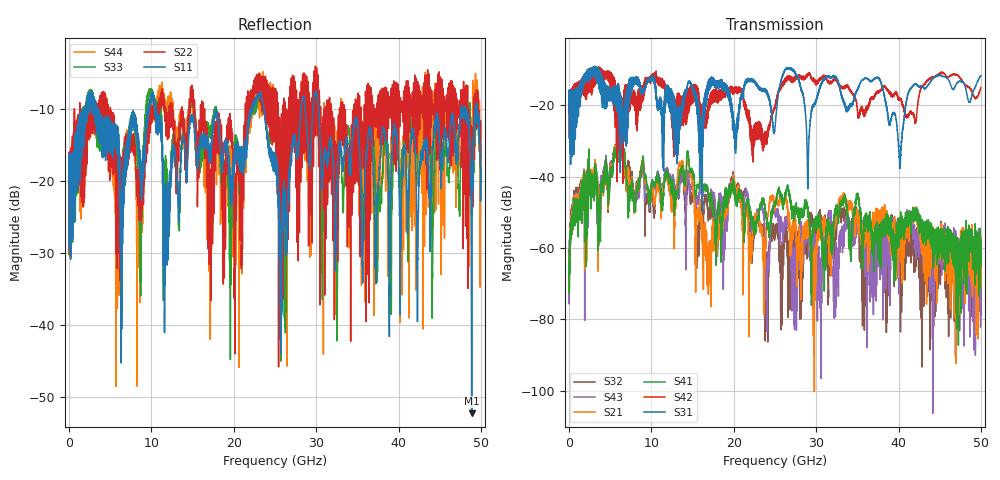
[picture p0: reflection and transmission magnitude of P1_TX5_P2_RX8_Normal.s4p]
!Keysight Technologies,N5225B,MY57041031,A.13.20.10
!Date: Friday, May 31, 2019 11:40:32
!Correction: S11(Full 4 Port(1,2,3,4))
!S12(Full 4 Port(1,2,3,4))
!S13(Full 4 Port(1,2,3,4))
!S14(Full 4 Port(1,2,3,4))
!S21(Full 4 Port(1,2,3,4))
!S22(Full 4 Port(1,2,3,4))
!S23(Full 4 Port(1,2,3,4))
!S24(Full 4 Port(1,2,3,4))
!S31(Full 4 Port(1,2,3,4))
!S32(Full 4 Port(1,2,3,4))
!S33(Full 4 Port(1,2,3,4))
!S34(Full 4 Port(1,2,3,4))
!S41(Full 4 Port(1,2,3,4))
!S42(Full 4 Port(1,2,3,4))
!S43(Full 4 Port(1,2,3,4))
!S44(Full 4 Port(1,2,3,4))
!S4P File: Measurements: <S11,S12,S13,S14>,
!<S21,S22,S23,S24>,
!<S31,S32,S33,S34>,
!<S41,S42,S43,S44>:
# Hz S  dB  R 50.0
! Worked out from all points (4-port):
!   5000 points, 10 MHz to 50 GHz, reference 50 ohm
!   strongest paths, dB at 10 MHz, 12.51 GHz, 25.01 GHz, 37.51 GHz, 50 GHz:
!     S31: -19.4, -23.1, -26.1, -12.3, -11.7
!     S42: -19.6, -22.3, -20.2, -16.3, -15.1
!     S41: -61.5, -41.8, -47.3, -56.3, -64.9
!     S21: -66.2, -45.6, -47.9, -51.7, -71.2
!     S43: -62.9, -40.5, -49.0, -65.2, -64.7
!     S32: -57.8, -44.3, -57.1, -57.2, -63.8
!   lowest |S11| = -52.2 dB at 48.88 GHz (marker M1), VSWR 1.00, Z = 49.8 + j0.0184 ohm
!   |S11| at or under -10 dB: 3.502 GHz to 9.556 GHz (6.054 GHz wide, 92.7 % of centre); 10.5 GHz to 22.11 GHz (11.6 GHz wide, 71.2 % of centre); 30.29 GHz to 47.6 GHz (17.3 GHz wide, 44.4 % of centre)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
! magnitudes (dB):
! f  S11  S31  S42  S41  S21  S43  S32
! 10 MHz  -19.9  -19.4  -19.6  -61.5  -66.2  -62.9  -57.8
! 6.34 GHz  -45.3  -20.2  -28.5  -31.3  -31.2  -31.2  -30.9
! 17.02 GHz  -15.6  -15.8  -18.2  -45.9  -62.1  -45.2  -49.3
! 19.88 GHz  -20.9  -21.8  -16.9  -40.7  -39.8  -39.9  -38.8
! 23.97 GHz  -12.9  -16.5  -29.7  -52.1  -53.3  -74.0  -68.7
! 48.88 GHz  -52.2  -17.6  -16.0  -58.6  -67.4  -63.3  -79.2
! 50 GHz  -18.1  -11.7  -15.1  -64.9  -71.2  -64.7  -63.8
